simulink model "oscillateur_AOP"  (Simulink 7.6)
settings: Solver=ode15s  StartTime=0.0  StopTime=100  RelTol=1e-3
libraries: fl_lib x6, nesl_utility x2, elec_lib x1

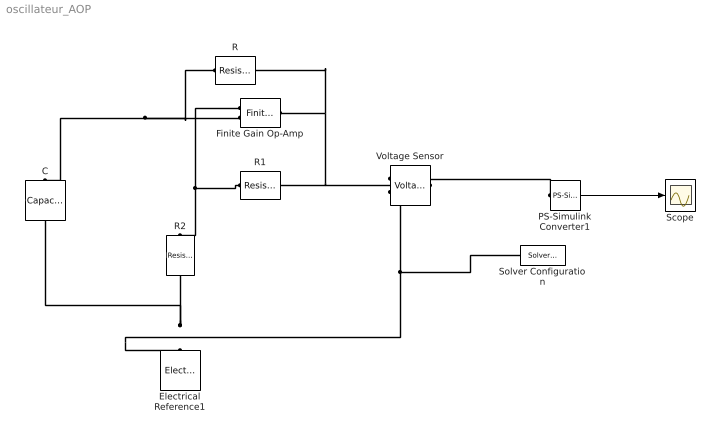
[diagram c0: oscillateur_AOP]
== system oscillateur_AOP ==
  C : fl_lib/Electrical/Electrical Elements/Capacitor  DialogController=NetworkEngine.DynNeDlgSource  SystemSampleTime=-1  c=1e-3 F  v0=0.1 V  r=1e-6 Ohm  g=0 1/Ohm  i_Log=off  v_Log=off  vc_Log=off  LocalVarNames=|i|v|vc  LocalVarDescs=|i|v|Internal variable for voltage across capacitor term  LocalVarLogging=[0 0 0]
  Electrical Reference1 : fl_lib/Electrical/Electrical Elements/Electrical Reference  DialogController=NetworkEngine.DynNeDlgSource  SystemSampleTime=-1  i_Log=off  LocalVarNames=|i  LocalVarDescs=|i  LocalVarLogging=0
  Finite Gain Op-Amp : elec_lib/Integrated Circuits/Finite Gain Op-Amp  DialogController=NetworkEngine.DynNeDlgSource  SystemSampleTime=-1  A=1000  Rin=1e+6 Ohm  Rout=100 Ohm  Vmin=-15 V  Vmax=15 V  LocalVarLogging=[]
  PS-Simulink Converter1 : nesl_utility/PS-Simulink Converter  DialogController=NetworkEngine.DynNeUtilDlgSource  SystemSampleTime=-1  PhysicalDomain=network_engine_domain  LeftPortType=input  RightPortType=output  SubClassName=ps_output  Unit=1  AffineConversion=off
  R : fl_lib/Electrical/Electrical Elements/Resistor  DialogController=NetworkEngine.DynNeDlgSource  SystemSampleTime=-1  R=1 kOhm  i_Log=off  v_Log=off  LocalVarNames=|i|v  LocalVarDescs=|i|v  LocalVarLogging=[0 0]
  R1 : fl_lib/Electrical/Electrical Elements/Resistor  DialogController=NetworkEngine.DynNeDlgSource  SystemSampleTime=-1  R=10 kOhm  i_Log=off  v_Log=off  LocalVarNames=|i|v  LocalVarDescs=|i|v  LocalVarLogging=[0 0]
  R2 : fl_lib/Electrical/Electrical Elements/Resistor  DialogController=NetworkEngine.DynNeDlgSource  SystemSampleTime=-1  R=10 kOhm  i_Log=off  v_Log=off  LocalVarNames=|i|v  LocalVarDescs=|i|v  LocalVarLogging=[0 0]
  Scope : Scope
  Solver Configuration : nesl_utility/Solver Configuration  DialogController=NetworkEngine.DynNeUtilDlgSource  SystemSampleTime=-1  PhysicalDomain=network_engine_domain  LeftPortType=input  RightPortType=generic  SubClassName=solver  Accelerate=off  Profile=off  ResidualTolerance=1e-9  MaxNonlinIter=12  MaxModeIter=2  DoFixedCost=off  UseLocalSampling=off  DoDC=off  LinearAlgebra=Sparse  LocalSolverSampleTime=.001  LocalSolverChoice=NE_BACKWARD_EULER_ADVANCER  UseLocalSolver=off
  Voltage Sensor : fl_lib/Electrical/Electrical Sensors/Voltage Sensor  DialogController=NetworkEngine.DynNeDlgSource  SystemSampleTime=-1  i1_Log=off  v1_Log=off  LocalVarNames=|i1|v1  LocalVarDescs=|i1|v1  LocalVarLogging=[0 0]
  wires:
  PS-Simulink Converter1/1 -> Scope/1
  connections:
  PS-Simulink Converter1/LConn1 -- Voltage Sensor/RConn1
  Finite Gain Op-Amp/LConn1 -- R1/RConn1 -- R2/LConn1
  Voltage Sensor/RConn2 -- R2/RConn1 -- C/LConn1 -- Electrical Reference1/LConn1 -- Solver Configuration/RConn1
  Finite Gain Op-Amp/RConn1 -- R1/LConn1 -- Voltage Sensor/LConn1 -- R/LConn1
  Finite Gain Op-Amp/LConn2 -- C/RConn1 -- R/RConn1
